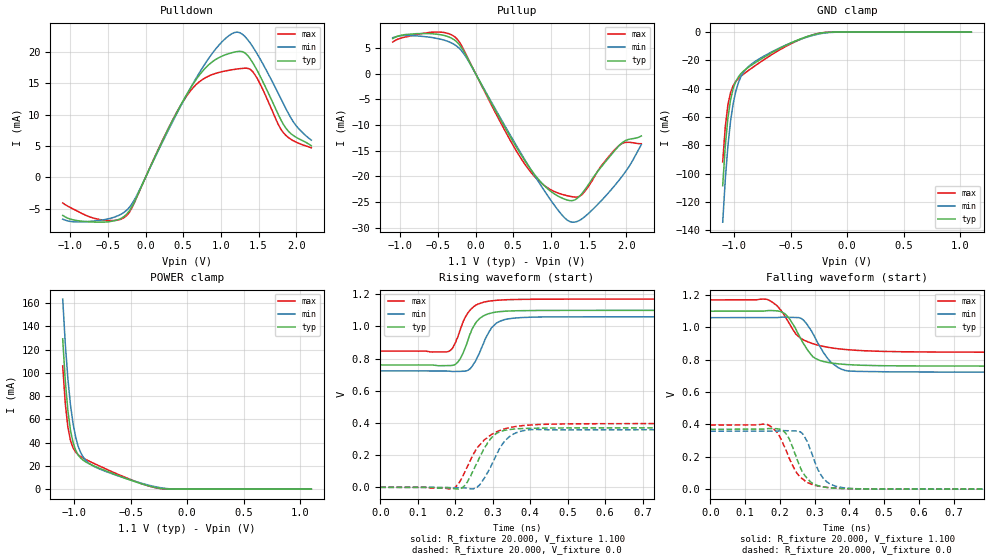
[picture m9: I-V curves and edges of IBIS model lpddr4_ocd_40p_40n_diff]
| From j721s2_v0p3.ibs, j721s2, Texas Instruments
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|   Model lpddr4_ocd_40p_40n_diff
[Model] lpddr4_ocd_40p_40n_diff
Model_type I/O
Polarity   Non-Inverting
Enable   Active-High
Vinl =  0.113V
Vinh =  0.253V
Vmeas =  0.183V
C_comp   1.480pF   1.310pF   1.728pF
[Model Spec]
Vinh   0.253V   0.247V   0.265V
Vinl   0.113V   0.107V   0.125V
Vmeas   0.183V   0.176V   0.195V
[Temperature Range]   25.000   0.125k   -40.000
[Voltage Range]   1.100V   1.060V   1.170V
[Pullup Reference]   1.100V   1.060V   1.170V
[Pulldown Reference]   0.0V   0.0V   0.0V
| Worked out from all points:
|   slope of the pulldown table from 0 to 0.165 V, typ, clamps not added: 38.6 ohm
|   slope of the pullup table from 0 to 0.165 V, typ, clamps not added: 36.5 ohm
|   GND clamp passes 1 mA (typ) near -0.25 V on its own axis
|   POWER clamp passes 1 mA (typ) near -0.26 V on its own axis
|   rising waveform, R_fixture 20.000, V_fixture 1.100: 20-80 % time 38.3ps typ, 42ps min, 38.6ps max; typ from 0.761 V to 1.1 V
|   rising waveform, R_fixture 20.000, V_fixture 0.0: 20-80 % time 50.5ps typ, 50.6ps min, 67.6ps max; typ from 0 V to 0.371 V
|   falling waveform, R_fixture 20.000, V_fixture 1.100: 20-80 % time 57.3ps typ, 58.2ps min, 76ps max; typ from 1.1 V to 0.761 V
|   falling waveform, R_fixture 20.000, V_fixture 0.0: 20-80 % time 45.8ps typ, 43.1ps min, 55.5ps max; typ from 0.371 V to 0 V
[Pulldown]
|Voltage   I(typ)   I(min)   I(max)
-1.1V     -6.056mA   -6.655mA   -4.075mA
-658mV    -7.127mA   -6.914mA   -6.587mA
-284mV    -6.208mA   -5.549mA   -6.391mA
-113mV    -2.983mA   -2.787mA   -3.073mA
295mV     7.517mA    7.322mA    7.635mA
567mV     13.62mA    13.58mA    13.31mA
839mV     17.92mA    18.95mA    16.13mA
1.179V    19.93mA    23.04mA    17.18mA
1.418V    18.32mA    20.86mA    16.88mA
1.826V    8.488mA    11.79mA    7.15mA
1.996V    6.386mA    8.256mA    5.615mA
2.2V      5.031mA    5.921mA    4.7mA
[Pullup]
|Voltage   I(typ)   I(min)   I(max)
-1.1V     6.815mA    6.988mA    6.146mA
-590mV    7.773mA    7.045mA    8.052mA
-249mV    6.184mA    5.339mA    6.801mA
-113mV    3.142mA    2.914mA    3.349mA
397mV     -10.68mA   -10.35mA   -11.3mA
669mV     -17.28mA   -17.12mA   -17.92mA
941mV     -22.2mA    -23.4mA    -22.08mA
1.247V    -24.7mA    -28.76mA   -23.85mA
1.418V    -23.22mA   -28.2mA    -23.46mA
1.69V     -17.76mA   -24.39mA   -17.55mA
1.928V    -13.68mA   -20.3mA    -13.72mA
2.2V      -12.13mA   -13.82mA   -13.64mA
[GND_clamp]
|Voltage   I(typ)   I(min)   I(max)
-1.1V     -108.4mA   -134.2mA   -91.64mA
-1.077V   -80.17mA   -103.9mA   -66.63mA
-1.054V   -60.68mA   -80.47mA   -51.43mA
-1.031V   -48.01mA   -63.16mA   -42.83mA
-1.008V   -40.05mA   -50.75mA   -37.96mA
-985mV    -35.04mA   -42.04mA   -34.98mA
-940mV    -29.42mA   -31.64mA   -31.22mA
-894mV    -26.11mA   -26.16mA   -28.35mA
-848mV    -23.5mA    -22.73mA   -25.7mA
-527mV    -8.739mA   -8.686mA   -9.514mA
-229mV    -630.6uA   -1.042mA   -565.7uA
1.1V      0A         0A         0A
[POWER_clamp]
|Voltage   I(typ)   I(min)   I(max)
-1.1V     129.2mA    163.4mA    105.9mA
-1.077V   92.86mA    124.8mA    73.4mA
-1.054V   67.3mA     94.73mA    53.17mA
-1.031V   50.48mA    72.25mA    41.67mA
-1.008V   39.92mA    56.03mA    35.37mA
-985mV    33.38mA    44.6mA     31.76mA
-963mV    29.31mA    36.69mA    29.53mA
-917mV    24.75mA    27.38mA    26.61mA
-871mV    22.09mA    22.57mA    24.31mA
-619mV    11.98mA    11.76mA    13.12mA
-229mV    602.7uA    1.183mA    400.7uA
1.1V      0A         0A         0A
[Ramp]
| variable   typ   min   max
dV/dt_r   0.222/50.795p   0.215/50.108p   0.238/67.157p
dV/dt_f   0.204/56.067p   0.202/57.835p   0.194/74.876p
R_load = 20.000
[Rising Waveform]
R_fixture= 20.000
V_fixture= 1.100
V_fixture_min= 1.060
V_fixture_max= 1.170
|time   V(typ)   V(min)   V(max)
0s        760.6mV    723.5mV    846.6mV
181ps     756.8mV    722.6mV    843.4mV
195ps     759.3mV    719.7mV    871.8mV
207ps     777.4mV    720.3mV    934.5mV
232ps     900.8mV    725.3mV    1.077V
247ps     992.8mV    758.5mV    1.117V
269ps     1.057V     859.4mV    1.146V
296ps     1.084V     989mV      1.159V
340ps     1.096V     1.046V     1.166V
3ns       1.1V       1.06V      1.17V
[Rising Waveform]
R_fixture= 20.000
V_fixture= 0.0
V_fixture_min= 0.0
V_fixture_max= 0.0
|time   V(typ)   V(min)   V(max)
0s        117.4uV    185.9uV    223.2uV
195ps     -6.581mV   -3.347mV   -7.704mV
223ps     4.764mV    -2.555mV   82.61mV
253ps     128mV      -6.308mV   222.8mV
275ps     232.9mV    46.41mV    286.6mV
307ps     330.9mV    187.4mV    341.7mV
326ps     350.4mV    268.6mV    359.7mV
345ps     359.5mV    316.3mV    370.9mV
408ps     367.4mV    359.4mV    388.7mV
3ns       370.5mV    358.4mV    396.6mV
[Falling Waveform]
R_fixture= 20.000
V_fixture= 1.100
V_fixture_min= 1.060
V_fixture_max= 1.170
|time   V(typ)   V(min)   V(max)
0s        1.1V       1.06V      1.17V
169ps     1.104V     1.06V      1.168V
193ps     1.102V     1.061V     1.131V
217ps     1.08V      1.063V     1.059V
259ps     934.3mV    1.058V     934.4mV
280ps     859.3mV    1.014V     910.2mV
301ps     808.9mV    935.8mV    894.7mV
345ps     780.6mV    788.4mV    874.4mV
405ps     768.6mV    729.1mV    860.3mV
3ns       760.6mV    723.5mV    846.6mV
[Falling Waveform]
R_fixture= 20.000
V_fixture= 0.0
V_fixture_min= 0.0
V_fixture_max= 0.0
|time   V(typ)   V(min)   V(max)
0s        370.5mV    358.4mV    396.6mV
166ps     374.5mV    358.4mV    398.3mV
192ps     373.6mV    358.9mV    350.8mV
216ps     348.5mV    361.7mV    247.8mV
242ps     226.3mV    360.2mV    121.3mV
259ps     131.7mV    354.7mV    75.39mV
278ps     68.06mV    299mV      44.83mV
316ps     17.81mV    94.55mV    16.85mV
360ps     5.949mV    19.01mV    6.393mV
3ns       117.5uV    185.8uV    223.1uV
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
